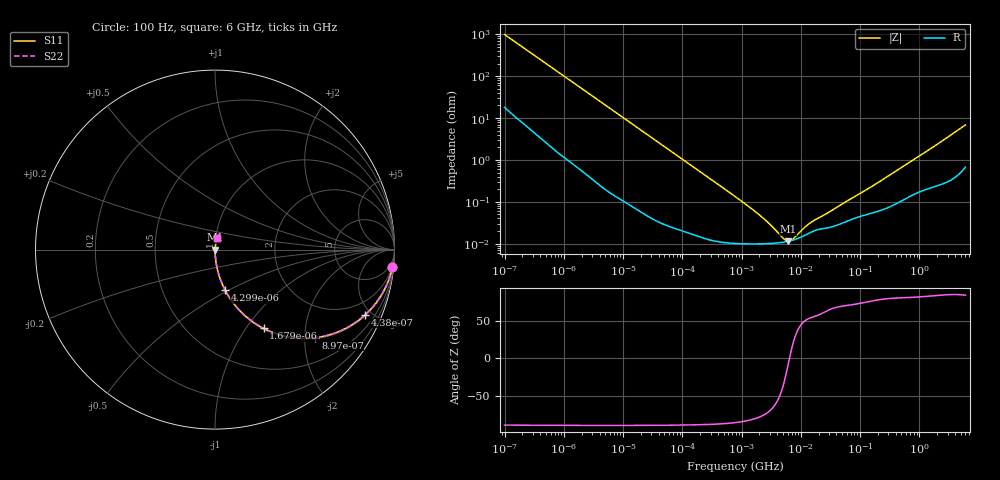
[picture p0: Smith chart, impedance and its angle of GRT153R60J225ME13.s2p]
!Murata Part Number: GRT153R60J225ME13
!These Parameters are Measured in Series Mode Connection
!Data Generated on Jun 19, 2026
!  o--ll--o
!Port1  Port2
!  o------o
!Operation Temp=25[degC], DC Bias Voltage=0[V]
!Freq. Start=100[Hz] Stop=6[GHz] 401[Steps]
# Hz S RI R 50
!Freq.(Hz) S11(Real) S11(Imag) S21(Real) S21(Imag) S12(Real) S12(Imag) S22(Real) S22(Imag)
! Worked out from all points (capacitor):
!   401 points, 100 Hz to 6 GHz, reference 50 ohm
!   read as one part in series: C = 1.6 uF near 109 Hz
!   lowest |Z| = 11.5 mohm at 6.075 MHz (marker M1)
!   series resonance near 6.431 MHz, so ESL is about 380 pH
!   S11 on the Smith chart (normalised r, x): 100 Hz: 1, -20; 438 Hz: 1.06, -4.59; 897 Hz: 1.03, -2.26; 1.679 kHz: 1.01, -1.21; 4.299 kHz: 1.00, -0.48; 6 GHz: 1.01, +0.14
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100  0.9882 -0.0992  0.0118 0.0992  0.0118 0.0992  0.9882 -0.0992
245  0.9406 -0.2291  0.0594 0.2291  0.0594 0.2291  0.9406 -0.2291
438  0.8374 -0.3625  0.1626 0.3625  0.1626 0.3625  0.8374 -0.3625
600  0.7365 -0.4345  0.2635 0.4345  0.2635 0.4345  0.7365 -0.4345
897  0.5591 -0.4908  0.4409 0.4908  0.4409 0.4908  0.5591 -0.4908
1227  0.4066 -0.4856  0.5934 0.4856  0.5934 0.4856  0.4066 -0.4856
1679  0.2702 -0.4386  0.7298 0.4386  0.7298 0.4386  0.2702 -0.4386
2008  0.2067 -0.3996  0.7933 0.3996  0.7933 0.3996  0.2067 -0.3996
2873  0.1143 -0.3131  0.8857 0.3131  0.8857 0.3131  0.1143 -0.3131
4299  0.0554 -0.224  0.9446 0.224  0.9446 0.224  0.0554 -0.224
11009  0.00956 -0.0923  0.9904 0.0923  0.9904 0.0923  0.00956 -0.0923
40335  0.000981 -0.0256  0.999 0.0256  0.999 0.0256  0.000981 -0.0256
774597  0.000102 -0.00134  0.9999 0.00134  0.9999 0.00134  0.000102 -0.00134
2074311  9.89e-05 -0.000454  0.9999 0.000454  0.9999 0.000454  9.89e-05 -0.000454
3103719  0.000101 -0.000259  0.9999 0.000259  0.9999 0.000259  0.000101 -0.000259
5079039  0.000108 -7.68e-05  0.9999 7.68e-05  0.9999 7.68e-05  0.000108 -7.68e-05
6075234  0.000113 -1.82e-05  0.9999 1.82e-05  0.9999 1.82e-05  0.000113 -1.82e-05
7266822  0.000121 3.91e-05  0.9999 -3.91e-05  0.9999 -3.91e-05  0.000121 3.91e-05
1.137099e7  0.000155 0.000181  0.9998 -0.000181  0.9998 -0.000181  0.000155 0.000181
1.555665e7  0.000193 0.000275  0.9998 -0.000275  0.9998 -0.000275  0.000193 0.000275
3.124326e8  0.000767 0.00423  0.9992 -0.00423  0.9992 -0.00423  0.000767 0.00423
6e9  0.0112 0.0669  0.9888 -0.0669  0.9888 -0.0669  0.0112 0.0669
